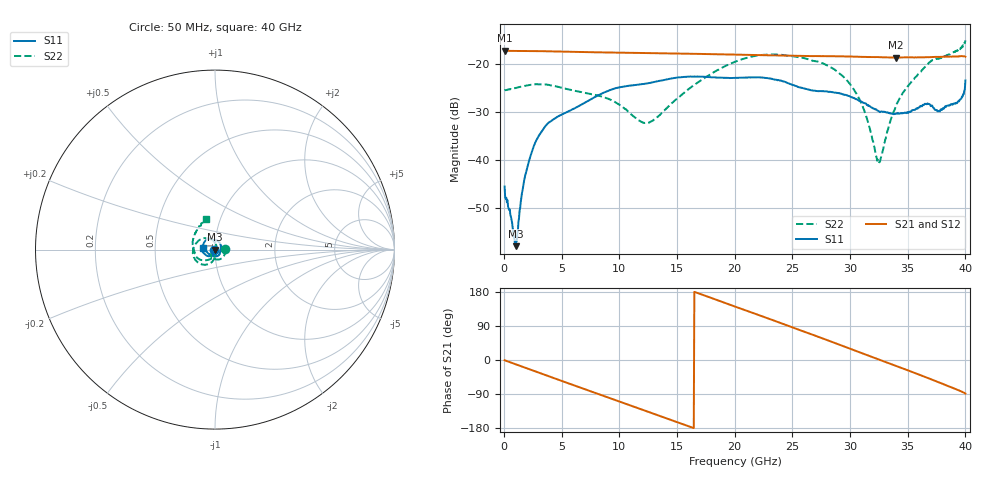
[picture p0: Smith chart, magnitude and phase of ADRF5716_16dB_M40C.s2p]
! Device: ADRF5716
! Description: 30GHz 2-Bit Digital Attenuator
! Frequency: 100 MHz – 30 GHz
! Ports:
! ATTIN  = Port 1
! ATTOUT = Port 2
! State: 16 dB Attenuation selected
! Supply Voltage:
! VDD  =  +3.30 Volts
! VSS  =  -3.30 Volts
! Control Voltages:
! D5 = 3.3V, D6 = 0V
! Temperature = -40 C
! Data: Data was collected using a calibrated network analyzer.
!  The reference plane is the package pins of ADRF5716 switch.
! Note: Analog Devices supplies this data as a sample of measured data for this product.
!  Your particular data for this product may vary.
!  Analog Devices reserves the right to change this data at anytime
# HZ S DB R 50
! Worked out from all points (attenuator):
!   800 points, 50 MHz to 40 GHz, reference 50 ohm
!   highest |S21| = -17.26 dB at 100 MHz (marker M1); lowest = -18.7 dB at 34 GHz (marker M2)
!   lowest |S11| = -57.8 dB at 1 GHz (marker M3), VSWR 1.00, Z = 49.9 - j0.0932 ohm
!   |S11| at or under -10 dB: start of sweep to end of sweep
!   |S22| runs from -40.6 to -15.1 dB; largest |S21 - S12| = 0
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5e7  -45.44 -143.7  -17.27 -0.6  -17.27 -0.6  -25.52 2.0
1e8  -47.75 174.1  -17.26 -1.2  -17.26 -1.2  -25.40 -0.3
1e9  -57.83 -133.3  -17.30 -11.2  -17.30 -11.2  -24.98 -11.7
1.85e9  -42.98 -70.6  -17.31 -20.5  -17.31 -20.5  -24.52 -25.3
2.8e9  -35.83 -83.2  -17.32 -31.1  -17.32 -31.1  -24.21 -42.0
3.9e9  -32.12 -101.1  -17.37 -43.3  -17.37 -43.3  -24.35 -61.5
6.75e9  -28.37 -121.2  -17.52 -74.2  -17.52 -74.2  -25.85 -98.4
9.4e9  -25.25 -138.5  -17.62 -103.1  -17.62 -103.1  -27.62 -124.0
1.205e10  -24.16 -156.6  -17.72 -131.8  -17.72 -131.8  -32.17 -119.5
1.34e10  -23.52 -163.3  -17.76 -146.6  -17.76 -146.6  -30.82 -97.8
2.005e10  -22.89 153.8  -18.05 140.7  -18.05 140.7  -19.51 -127.4
2.3e10  -23.01 129.6  -18.19 108.4  -18.19 108.4  -18.03 -160.6
2.67e10  -25.47 98.2  -18.36 67.3  -18.36 67.3  -19.28 159.0
3.025e10  -27.01 51.2  -18.47 26.9  -18.47 26.9  -24.98 106.1
3.125e10  -28.12 34.3  -18.54 15.4  -18.54 15.4  -29.81 82.3
3.245e10  -29.74 15.2  -18.58 1.8  -18.58 1.8  -40.25 -3.2
3.335e10  -30.12 1.9  -18.64 -8.4  -18.64 -8.4  -32.93 -75.2
3.4e10  -30.31 -7.4  -18.67 -15.6  -18.67 -15.6  -28.63 -94.7
3.645e10  -28.35 -59.3  -18.60 -44.1  -18.60 -44.1  -20.72 -140.1
3.78e10  -29.83 -92.9  -18.53 -60.2  -18.53 -60.2  -18.80 -172.1
3.945e10  -27.76 -143.9  -18.39 -80.3  -18.39 -80.3  -17.07 142.7
4e10  -23.42 173.8  -18.48 -88.4  -18.48 -88.4  -15.11 106.4
